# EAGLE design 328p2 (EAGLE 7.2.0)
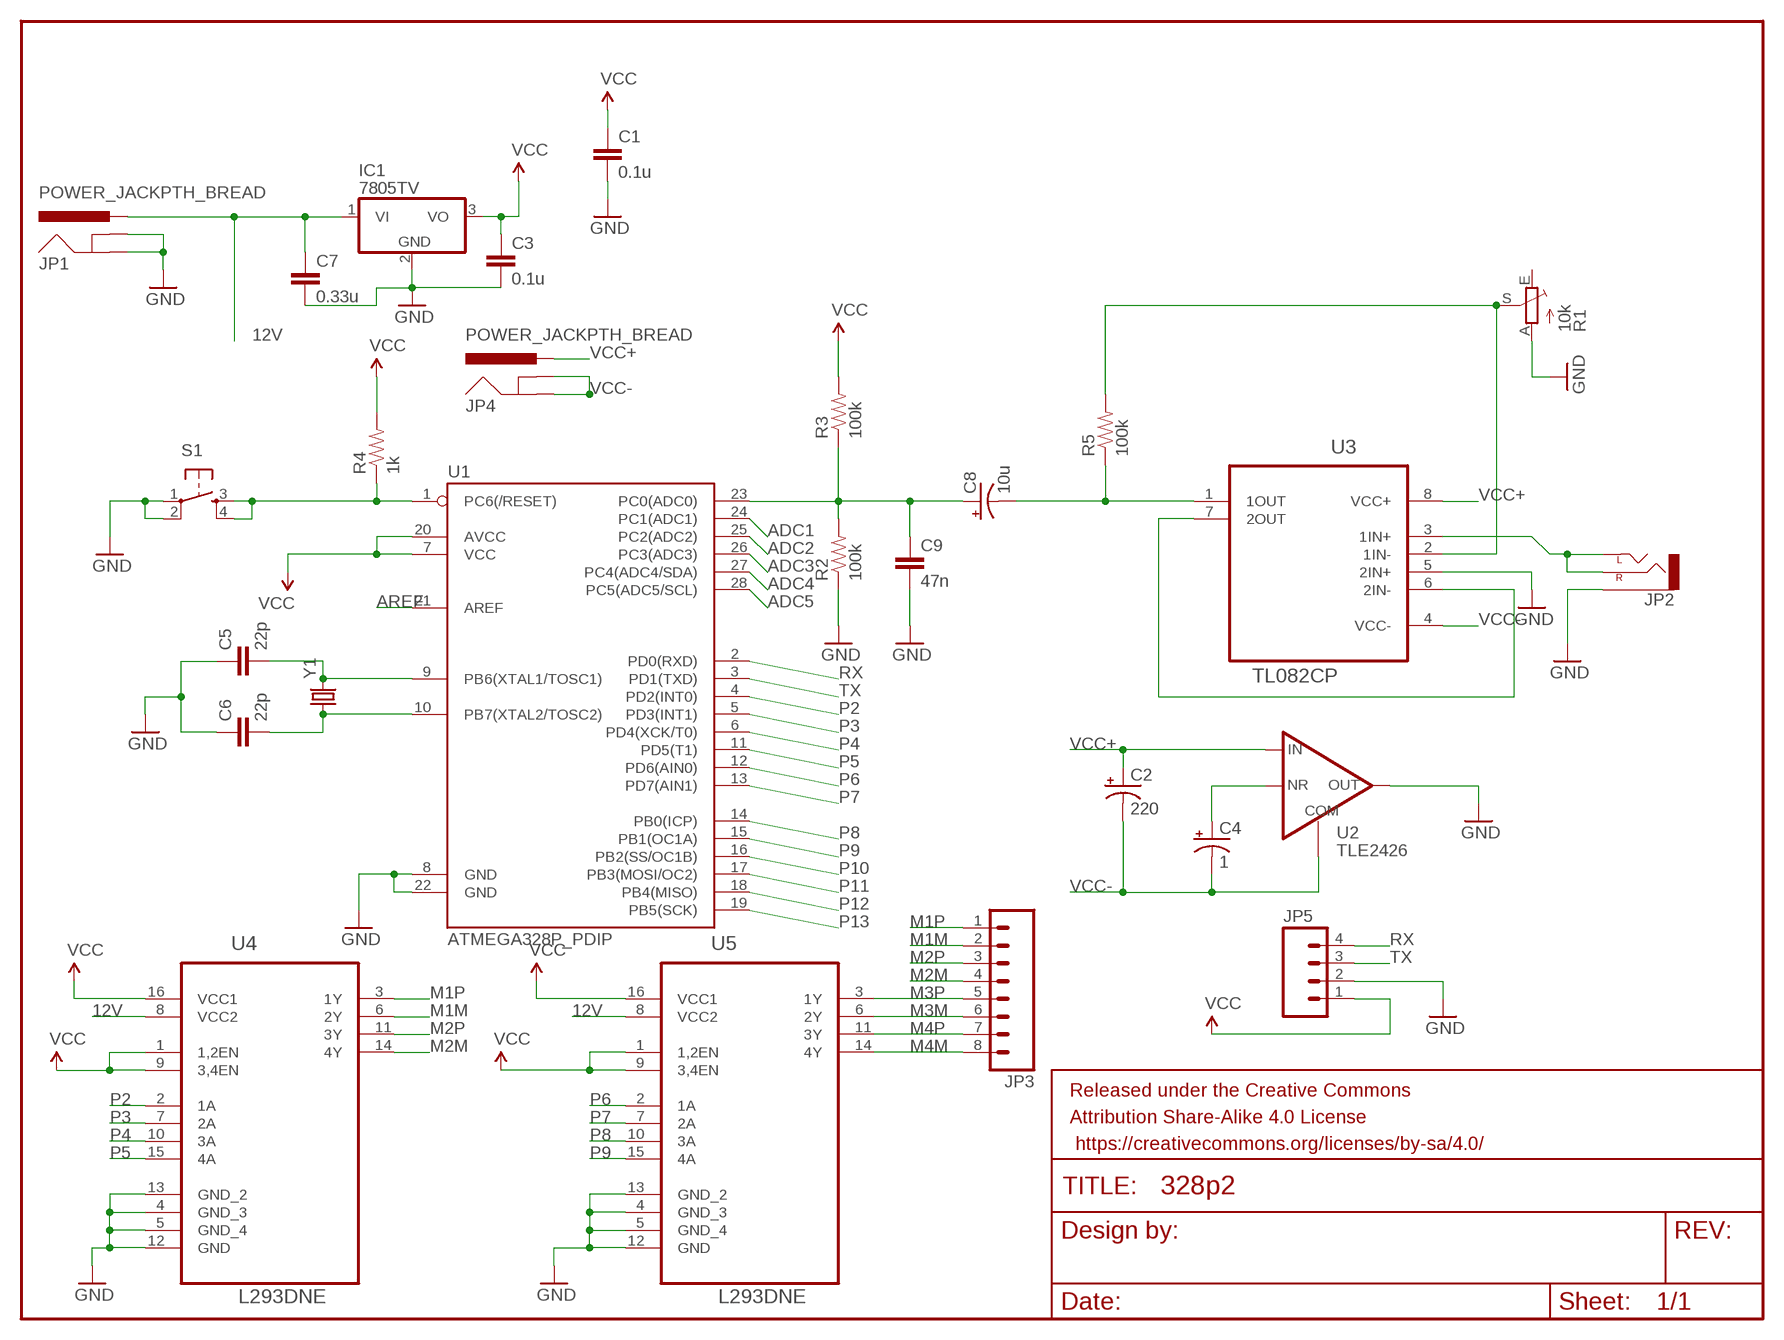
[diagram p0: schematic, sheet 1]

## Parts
C1  0.1u  CAP_  [AXIAL-5MM]
C2  220  CAP_POLPTH2  [CPOL-RADIAL-10UF-25V]
C3  0.1u  CAP_  [AXIAL-5MM]
C4  1  CAP_POLPTH1  [CPOL-RADIAL-100UF-25V]
C5  22p  CAP_  [AXIAL-5MM]
C6  22p  CAP_  [AXIAL-5MM]
C7  0.33u  CAP_  [AXIAL-5MM]
C8  10u  CAP_POLPTH1  [CPOL-RADIAL-100UF-25V]
C9  47n  CAP_  [AXIAL-5MM]
FRAME1  FRAME-LETTER  [CREATIVE_COMMONS]
IC1  7805TV  [TO220V]
JP1  POWER_JACKPTH_BREAD  [POWER_JACK_PTH_BREAD]
JP2  AUDIO-JACKPTH  [AUDIO-JACK]
JP3  M08  [1X08_ROUND]
JP4  POWER_JACKPTH_BREAD  [POWER_JACK_PTH_BREAD]
JP5  M04PTH  [1X04]
R1  10k  TRIM_EU-B25P  [B25P]
R2  100k  RESISTORPTH-1/4W  [AXIAL-0.4]
R3  100k  RESISTORPTH-1/4W  [AXIAL-0.4]
R4  1k  RESISTORPTH-1/4W  [AXIAL-0.4]
R5  100k  RESISTORPTH-1/4W  [AXIAL-0.4]
S1  TAC_SWITCHPTH  [TACTILE-PTH]
U1  ATMEGA328P_PDIP  [DIL28-3]
U2  TLE2426  TLE2426_RAIL_SPLITTER  [SO08]
U3  TL082CP  [DIP254P762X508-8]
U4  L293DNE  [DIP254P762X508-16]
U5  L293DNE  [DIP254P762X508-16]
Y1  CRYSTALHC49US  [HC49US]

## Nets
12V: C7.P$1 IC1.1(VI) JP1.PWR U4.8(VCC2) U5.8(VCC2)
ADC1: U1.24(PC1(ADC1))
ADC2: U1.25(PC2(ADC2))
ADC3: U1.26(PC3(ADC3))
ADC4: U1.27(PC4(ADC4/SDA))
ADC5: U1.28(PC5(ADC5/SCL))
AREF: U1.21(AREF)
GND: C1.P$2 C3.P$2 C5.P$1 C6.P$1 C7.P$2 C9.P$2 IC1.2(GND) JP1.GND JP1.GNDBREAK JP2.SLEEVE JP5.2 R1.A R2.P$1 S1.1 S1.2 U1.8(GND) U1.22(GND) U2.1(OUT) U3.5(2IN+) U4.4(GND_3) U4.5(GND_4) U4.12(GND) U4.13(GND_2) U5.4(GND_3) U5.5(GND_4) U5.12(GND) U5.13(GND_2)
M1M: JP3.2 U4.6(2Y)
M1P: JP3.1 U4.3(1Y)
M2M: JP3.4 U4.14(4Y)
M2P: JP3.3 U4.11(3Y)
M3M: JP3.6 U5.6(2Y)
M3P: JP3.5 U5.3(1Y)
M4M: JP3.8 U5.14(4Y)
M4P: JP3.7 U5.11(3Y)
N$1: R4.P$1 S1.3 S1.4 U1.1(PC6(/RESET))
N$2: C5.P$2 U1.9(PB6(XTAL1/TOSC1)) Y1.2
N$3: C6.P$2 U1.10(PB7(XTAL2/TOSC2)) Y1.1
N$4: R1.S R5.P$2 U3.2(1IN-)
N$5: C8.1(+) C9.P$1 R2.P$2 R3.P$1 U1.23(PC0(ADC0))
N$6: C8.2(-) R5.P$1 U3.1(1OUT)
N$7: JP2.RING(RIGHT) JP2.TIP(LEFT) U3.3(1IN+)
N$8: U3.6(2IN-) U3.7(2OUT)
N$9: C4.1(+) U2.8(NR)
P2: U1.4(PD2(INT0)) U4.2(1A)
P3: U1.5(PD3(INT1)) U4.7(2A)
P4: U1.6(PD4(XCK/T0)) U4.10(3A)
P5: U1.11(PD5(T1)) U4.15(4A)
P6: U1.12(PD6(AIN0)) U5.2(1A)
P7: U1.13(PD7(AIN1)) U5.7(2A)
P8: U1.14(PB0(ICP)) U5.10(3A)
P9: U1.15(PB1(OC1A)) U5.15(4A)
P10: U1.16(PB2(SS/OC1B))
P11: U1.17(PB3(MOSI/OC2))
P12: U1.18(PB4(MISO))
P13: U1.19(PB5(SCK))
RX: JP5.4 U1.2(PD0(RXD))
TX: JP5.3 U1.3(PD1(TXD))
VCC: C1.P$1 C3.P$1 IC1.3(VO) JP5.1 R3.P$2 R4.P$2 U1.7(VCC) U1.20(AVCC) U4.1(1,2EN) U4.9(3,4EN) U4.16(VCC1) U5.1(1,2EN) U5.9(3,4EN) U5.16(VCC1)
VCC+: C2.1(+) JP4.PWR U2.3(IN) U3.8(VCC+)
VCC-: C2.2(-) C4.2(-) JP4.GND JP4.GNDBREAK U2.2(COM) U3.4(VCC-)
Unconnected: R1.E

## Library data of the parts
C1 C3 C5-C7 C9 = SparkFun-Capacitors:CAP: Capacitor
C2 C4 C8 = SparkFun-Passives:CAP_POL: Capacitor Polarized
FRAME1 = SparkFun-Aesthetics:FRAME-LETTER: Schematic Frame; DESIGNER: NAME; VERSION: v01
IC1 = linear:78*: Positive VOLTAGE REGULATOR Source: http://cache.national.com/ds/LM/LM78L05.pdf http://www.fairchildsemi.com/ds/LM/LM7805.pdf
JP1 JP4 = SparkFun-Connectors:POWER_JACK: Power Jack This is the standard 5.5mm barrel jack for power. The PTH is the most common, proven, reliable, footprint. The Slot footprint only works if the mill layer is transmitted to the PCB fab house so be warned. Mating wall wart : TOL-00298 (and others); PROD_ID: PRT-10811
JP2 = SparkFun-Connectors:AUDIO-JACK: 3.5mm Audio Jack Simple 3.5mm common PCB mount audio jack. Variant PTH is our storefront SKU PRT-08032
JP3 = SparkFun-Connectors:M08: Header 8 Standard 8-pin 0.1" header. Use with straight break away headers (SKU : PRT-00116), right angle break away headers (PRT-00553), swiss pins (PRT-00743), machine pins (PRT-00117), and female headers (PRT-00115).
JP5 = SparkFun-Connectors:M04: Header 4 Standard 4-pin 0.1" header. Use with straight break away headers (SKU : PRT-00116), right angle break away headers (PRT-00553), swiss pins (PRT-00743), machine pins (PRT-00117), and female headers (PRT-00115). Molex polarized connector foot print use with SKU : PRT-08231 with associated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
R1 = pot:TRIM_EU-: POTENTIOMETER
R2-R5 = SparkFun-Resistors:RESISTOR: Resistor
S1 = SparkFun-Retired:TAC_SWITCH: Momentary Switch Button commonly used for reset or general input. Spark Fun Electronics SKU : COM-00097 SMT- SWCH-08247
U1 = SparkFun-DigitalIC:ATMEGA328P_PDIP: uC used in the Arduino 32kb flash, 1k EEPROM, 2k SRAM This is the through-hole version of this chip.
U2 = SparkFun-PowerIC:TLE2426_RAIL_SPLITTER; PROD_ID: VREG-12334
U3 = Texas Instruments_By_element14_Batch_1:TL082CP: OPERATIONAL AMPLIFIER; MPN: TL082CP; OC_FARNELL: 1106017; OC_NEWARK: 60K6991; PACKAGE: PDIP; SUPPLIER: Texas Instruments
U4 U5 = Texas Instruments_By_element14_Batch_1:L293DNE: QUADRUPLE HALF-H DRIVERS; MPN: L293DNE; OC_FARNELL: 1470423; OC_NEWARK: 06F9523; PACKAGE: PDIP-16; SUPPLIER: Texas Instruments
Y1 = SparkFun-FreqCtrl:CRYSTAL: Various standard crystals. Proven footprints.

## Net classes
0 default: clearance 0.205 mm

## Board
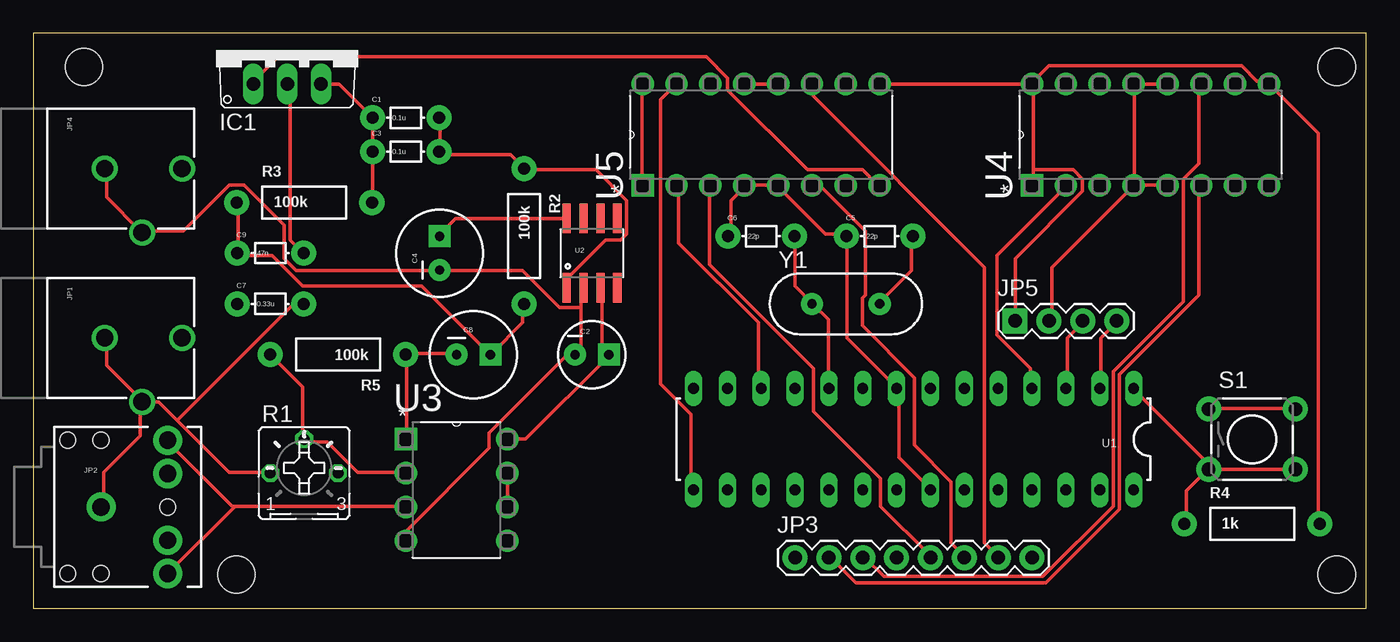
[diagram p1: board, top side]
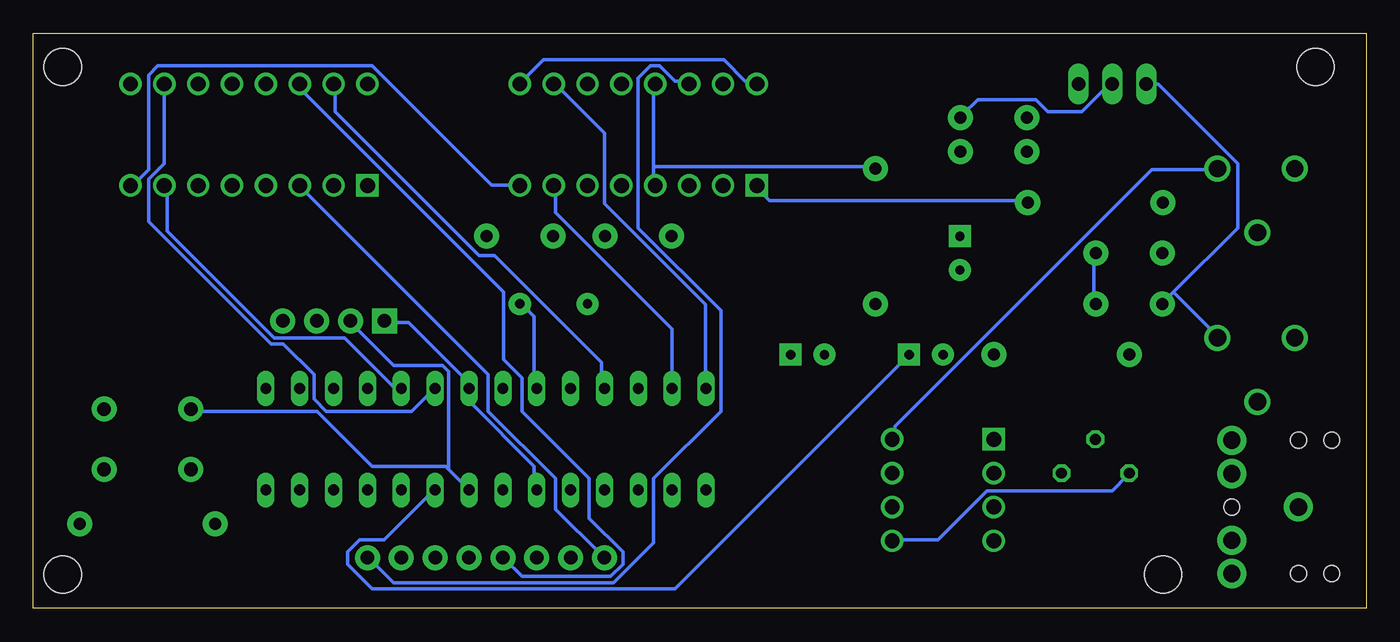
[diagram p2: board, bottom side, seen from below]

Size 100 x 43.17 mm. Coordinates in mm from the lower left corner, seen from the top.
Outline: 0,0 100,0 100,43.17 0,43.17 0,0
Copper layers (1*16): Top 0.035mm / dielectric 1.5mm / Bottom 0.035mm
Design rules "default": minimum track width 10mil, minimum drill 24mil, track to track 8mil, track to pad 8mil, pad to pad 8mil, via to via 8mil, smd to smd 8mil, copper to edge 40mil, drill to drill 8mil, minimum pad ring 10mil, minimum via ring 8mil, stop-mask expansion 4mil, vias tented up to drill 0mil, thermal gap 10mil
Holes 2.8 mm at 3.81,40.64 97.79,40.64 97.79,2.54 15.24,2.54

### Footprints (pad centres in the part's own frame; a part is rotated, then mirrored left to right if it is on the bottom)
AXIAL-5MM = drill 0.9 pad 1.88: P$1 -2.5,0; P$2 2.5,0
CPOL-RADIAL-10UF-25V = drill 0.7 pad 1.651 square: 1 1.27,0 | drill 0.7 pad 1.651: 2 -1.27,0
CPOL-RADIAL-100UF-25V = drill 0.7 pad 1.651 square: 1 1.27,0 | drill 0.7 pad 1.651: 2 -1.27,0
TO220V = drill 1.016 long: 1 -2.54,-2.54; 2 0,-2.54; 3 2.54,-2.54
POWER_JACK_PTH_BREAD = drill 1.3: GND 0,7.9; GNDBREAK 4.8,10.7; PWR 0,13.7
AUDIO-JACK = drill 1.3 pad 2.184: RING 5,5; RSH 5,2.5; SLEEVE 0,0; TIP 5,-5; TSH 5,-2.5 | hole 1.2: 0,5; -2.5,5; -2.5,-5; 0,-5; 5,0
1X08_ROUND = drill 1.016 pad 1.88: 1 0,0; 2 2.54,0; 3 5.08,0; 4 7.62,0; 5 10.16,0; 6 12.7,0; 7 15.24,0; 8 17.78,0
1X04 = drill 1.016 pad 1.88 square: 1 0,0 | drill 1.016 pad 1.88: 2 2.54,0; 3 5.08,0; 4 7.62,0
B25P = drill 0.813 octagon: A -2.54,0; E 2.54,0; S 0,2.54
AXIAL-0.4 = drill 0.9 pad 1.88: P$1 -5.08,0; P$2 5.08,0
TACTILE-PTH = drill 1.016 pad 1.88: 1 -3.251,2.261; 2 3.251,2.261; 3 -3.251,-2.261; 4 3.251,-2.261
DIL28-3 = drill 0.813 long: 1 -16.51,-3.81; 2 -13.97,-3.81; 3 -11.43,-3.81; 4 -8.89,-3.81; 5 -6.35,-3.81; 6 -3.81,-3.81; 7 -1.27,-3.81; 8 1.27,-3.81; 9 3.81,-3.81; 10 6.35,-3.81; 11 8.89,-3.81; 12 11.43,-3.81; 13 13.97,-3.81; 14 16.51,-3.81; 15 16.51,3.81; 16 13.97,3.81; 17 11.43,3.81; 18 8.89,3.81; 19 6.35,3.81; 20 3.81,3.81; 21 1.27,3.81; 22 -1.27,3.81; 23 -3.81,3.81; 24 -6.35,3.81; 25 -8.89,3.81; 26 -11.43,3.81; 27 -13.97,3.81; 28 -16.51,3.81
SO08 = smd 0.61 x 2.21: 1 -1.905,-2.616; 2 -0.635,-2.616; 3 0.635,-2.616; 4 1.905,-2.616; 5 1.905,2.616; 6 0.635,2.616; 7 -0.635,2.616; 8 -1.905,2.616
DIP254P762X508-8 = drill 1.118 square: 1 -7.62,7.62 | drill 1.118: 2 -7.62,5.08; 3 -7.62,2.54; 4 -7.62,0; 5 0,0; 6 0,2.54; 7 0,5.08; 8 0,7.62
DIP254P762X508-16 = drill 1.118 square: 1 -7.62,17.78 | drill 1.118: 2 -7.62,15.24; 3 -7.62,12.7; 4 -7.62,10.16; 5 -7.62,7.62; 6 -7.62,5.08; 7 -7.62,2.54; 8 -7.62,0; 9 0,0; 10 0,2.54; 11 0,5.08; 12 0,7.62; 13 0,10.16; 14 0,12.7; 15 0,15.24; 16 0,17.78
HC49US = drill 0.7 pad 1.651: 1 -2.54,0; 2 2.54,0

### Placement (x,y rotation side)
C1  27.94,36.83 0 top
C2  41.91,19.05 0 top
C3  27.94,34.29 0 top
C4  30.48,26.67 90 top
C5  63.5,27.94 0 top
C6  54.61,27.94 0 top
C7  17.78,22.86 0 top
C8  33.02,19.05 0 top
C9  17.78,26.67 0 top
FRAME1  not placed on the board
IC1  19.05,41.91 0 top
JP1  -2.54,20.32 270 top
JP2  5.08,7.62 0 top
JP3  57.15,3.81 0 top
JP4  -2.54,33.02 270 top
JP5  73.66,21.59 0 top
R1  20.32,10.16 0 top
R2  36.83,27.94 270 top
R3  20.32,30.48 0 top
R4  91.44,6.35 0 top
R5  22.86,19.05 180 top
S1  91.44,12.7 0 top
U1  66.04,12.7 180 top
U2  41.91,26.67 0 top
U3  35.56,5.08 0 top
U4  92.71,39.37 90 top
U5  63.5,39.37 90 top
Y1  60.96,22.86 0 top

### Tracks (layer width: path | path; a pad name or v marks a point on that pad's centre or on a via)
12V
  Top 0.254: IC1.1 16.52,39.58 18.36,41.42 50.49,41.42 52.1,39.81 52.1,38.89 58.06,32.93 62.19,32.93 63.34,31.78 U5.8
  Bottom 0.254: 14.46,23.75 15.15,23.06 C7.P$1 | 14.46,23.75 9.64,28.57 9.64,33.38 15.61,39.35 16.29,39.35 IC1.1 | 14.46,23.75 11.24,20.53 JP1.PWR | U5.8 63.57,31.78 65.64,31.78 74.59,40.73 90.65,40.73 91.34,40.04 91.34,32.93 92.49,31.78 U4.8
GND
  Top 0.254: IC1.2 19.28,39.35 19.28,27.65 20.2,26.73 C9.P$2 | C1.P$2 30.52,36.83 30.52,34.3 C3.P$2 30.52,34.07 35.8,34.07 36.72,33.15 R2.P$1 36.95,32.93 42.23,32.93 44.52,30.63 44.52,28.11 44.06,27.65 42.92,27.65 40.16,24.89 40.16,24.2 U2.1 | 10.79,14.11 9.41,15.48 8.26,15.48 JP1.GNDBREAK | 10.79,14.11 14.69,10.21 17.67,10.21 R1.A | JP1.GND 5.51,20.3 5.51,18.24 8.03,15.71 JP1.GNDBREAK | JP2.SLEEVE 5.28,7.68 5.28,10.21 8.03,12.96 8.03,15.48 JP1.GNDBREAK | 10.79,14.11 19.51,22.83 20.2,22.83 C7.P$2 | 82.62,39.35 84.92,39.35 U4.12 | 82.62,31.78 84.92,31.78 U4.5 | JP5.2 76.42,21.68 76.42,25.58 82.39,31.55 U4.4 82.62,31.78 | 82.62,31.78 82.62,39.35 | 82.62,39.35 U4.13 | U5.13 53.47,39.35 55.77,39.35 U5.12 | C6.P$1 52.33,28.11 52.33,30.63 53.24,31.55 U5.4 53.47,31.78 55.77,31.78 U5.5 56,31.55 59.44,28.11 60.82,28.11 C5.P$1 61.05,27.88 61.05,20.3 64.72,16.63 U1.8 64.95,16.4 64.95,11.35 67.24,9.06 U1.22 | S1.1 88.36,15.02 94.55,15.02 S1.2
  Bottom 0.254: C7.P$2 20.43,23.06 20.43,26.5 C9.P$2 | IC1.2 19.28,39.35 21.34,37.29 23.87,37.29 24.79,38.2 29.15,38.2 30.29,37.06 C1.P$2 | U3.5 35.34,5.16 32.13,5.16 28.46,8.83 19.05,8.83 17.9,9.97 R1.A | 53.47,33.15 53.47,31.78 U5.4 | 53.47,33.15 53.47,39.35 U5.13 | 68.85,10.43 67.47,9.06 U1.22 | 68.85,10.43 69.08,10.66 74.59,10.66 78.72,14.8 88.13,14.8 S1.1 | 68.85,10.43 68.85,17.78 69.31,18.24 72.98,18.24 76.19,21.45 JP5.2 | 53.47,33.15 36.95,33.15 R2.P$1
M1M
  Top 0.254: U4.6 87.44,31.55 87.44,23.52 81.47,17.55 81.47,7.45 75.97,1.94 61.74,1.94 59.9,3.78 JP3.2
M1P
  Bottom 0.254: U4.3 79.87,31.55 65.87,17.55 65.87,14.8 60.82,9.75 60.82,7.45 57.38,4.01 JP3.1
M2M
  Bottom 0.254: U4.14 79.87,39.35 79.87,38.89 64.72,23.75 64.72,18.7 63.34,17.32 63.34,14.8 58.29,9.75 58.29,6.76 55.77,4.24 55.77,3.32 56.69,2.4 63.34,2.4 64.72,3.78 JP3.4
M2P
  Top 0.254: U4.11 87.44,39.35 87.44,33.38 86.29,32.24 86.29,23.06 81.01,17.78 81.01,7.68 75.73,2.4 63.8,2.4 62.42,3.78 JP3.3
M3M
  Top 0.254: U5.6 58.52,31.55 59.21,31.55 62.42,28.34 62.42,23.52 62.19,23.29 62.19,21.22 66.1,17.32 66.1,12.27 68.85,9.52 68.85,4.93 69.77,4.01 JP3.6
M3P
  Top 0.254: U5.3 50.72,31.55 50.72,25.81 58.52,18.01 58.52,14.8 63.57,9.75 63.57,7.68 67.24,4.01 JP3.5
M4M
  Bottom 0.254: U5.14 50.95,39.58 51.87,39.58 53.01,40.73 53.7,40.73 54.62,39.81 54.62,28.57 48.42,22.37 48.42,14.8 53.47,9.75 53.47,4.93 56.46,1.94 72.98,1.94 74.82,3.78 JP3.8
M4P
  Top 0.254: U5.11 58.52,39.35 58.52,38.43 71.37,25.58 71.37,4.93 72.29,4.01 JP3.7
N$1
  Top 0.254: U1.1 82.62,16.4 88.36,10.66 S1.3 | R4.P$1 86.52,6.53 86.52,8.83 88.13,10.43 S1.3 | S1.4 94.55,10.43 88.36,10.43 S1.3
N$2
  Top 0.254: C5.P$2 65.87,27.88 65.87,25.35 63.57,23.06 Y1.2
  Bottom 0.254: U1.9 62.42,16.63 62.42,21.91 63.34,22.83 Y1.2
N$3
  Top 0.254: U1.10 59.67,16.63 59.67,21.68 58.52,22.83 Y1.1 58.29,23.06 57.15,24.2 57.15,27.88 C6.P$2
N$4
  Top 0.254: R5.P$2 17.9,18.93 20.2,16.63 20.2,12.73 R1.S 20.43,12.5 22.03,12.5 24.33,10.21 27.77,10.21 U3.2
N$5
  Top 0.254: R3.P$1 15.38,30.4 15.38,26.73 C9.P$1 15.38,26.5 17.9,26.5 20.2,24.2 29.15,24.2 34.2,19.16 C8.1 34.42,19.16 36.72,21.45 36.72,22.83 R2.P$2
  Bottom 0.254: U1.23 70,8.83 73.67,5.16 75.5,5.16 76.42,4.24 76.42,3.32 74.59,1.48 51.87,1.48 34.42,18.93 C8.1
N$6
  Top 0.254: C8.2 31.67,19.16 28,19.16 R5.P$1 28,18.93 28,12.73 U3.1
N$7
  Top 0.254: 15.15,7.68 14.92,7.68 10.1,12.5 JP2.RING | 15.15,7.68 27.77,7.68 U3.3 | 15.15,7.68 10.1,2.63 JP2.TIP
N$8
  Top 0.254: U3.6 35.57,7.68 35.57,9.97 U3.7
N$9
  Top 0.254: U2.8 39.93,29.25 31.67,29.25 30.52,28.11 C4.1
P2
  Top 0.254: U1.4 74.82,16.63 74.82,18.01 72.29,20.53 72.29,26.5 77.34,31.55 U4.2
P3
  Bottom 0.254: U1.5 72.52,16.63 72.98,16.63 76.65,20.3 81.93,20.3 89.96,28.34 89.96,31.55 U4.7
P4
  Bottom 0.254: U1.6 70,16.4 71.6,14.8 78.03,14.8 78.95,15.71 78.95,17.55 81.24,19.84 82.16,19.84 91.34,29.02 91.34,32.24 90.19,33.38 90.19,39.35 U4.10
P5
  Bottom 0.254: U1.11 57.38,16.63 57.38,18.47 65.41,26.5 66.56,26.5 77.34,37.29 77.34,39.35 U4.15
P6
  Top 0.254: U1.12 54.39,16.63 54.39,21.45 48.42,27.42 48.42,31.55 U5.2
P7
  Bottom 0.254: U1.13 52.1,16.63 52.1,20.99 60.82,29.71 60.82,31.55 U5.7
P8
  Bottom 0.254: U1.14 49.57,16.63 49.57,22.83 57.15,30.4 57.15,35.68 60.82,39.35 U5.10
P9
  Top 0.254: U1.15 49.34,9.06 49.34,14.57 47.05,16.86 47.05,38.2 48.2,39.35 U5.15
RX
  Top 0.254: U1.2 80.1,16.63 80.1,20.3 81.24,21.45 JP5.4
TX
  Top 0.254: U1.3 77.57,16.63 77.57,20.3 78.72,21.45 JP5.3
VCC
  Top 0.254: R3.P$2 25.47,30.63 25.47,34.07 C3.P$1 25.47,34.3 25.47,36.83 C1.P$1 25.25,37.06 22.95,39.35 21.8,39.35 IC1.3 | U5.1 45.67,31.78 45.67,39.35 U5.16 | U5.9 63.57,39.35 74.82,39.35 U4.16 | 75.05,32.93 75.05,39.35 U4.16 | 75.05,32.93 75.05,31.78 U4.1 | U4.16 75.05,39.58 76.19,40.73 90.65,40.73 91.8,39.58 92.49,39.58 U4.9 92.72,39.35 96.39,35.68 96.39,6.53 R4.P$2 | 75.05,32.93 78.03,32.93 78.72,32.24 78.72,31.32 73.67,26.27 73.67,21.68 JP5.1
  Bottom 0.254: U1.20 62.42,9.06 62.42,10.66 67.24,15.48 67.24,16.4 U1.7 67.47,16.63 67.47,17.09 71.83,21.45 73.44,21.45 JP5.1 | U5.16 45.9,39.58 46.59,39.58 48.2,41.19 61.74,41.19 63.34,39.58 U5.9 | R3.P$2 25.47,30.63 44.75,30.63 45.67,31.55 U5.1
VCC+
  Top 0.254: U2.3 42.69,23.98 42.69,19.61 43.15,19.16 C2.1 43.15,18.93 36.95,12.73 35.57,12.73 U3.8
  Bottom 0.254: JP4.PWR 11.24,32.93 16.07,32.93 35.34,13.65 35.34,12.73 U3.8
VCC-
  Top 0.254: JP4.GND 5.51,32.93 5.51,30.86 8.03,28.34 JP4.GNDBREAK 8.26,28.34 11.24,28.34 14.69,31.78 15.84,31.78 18.82,28.79 18.82,26.27 19.74,25.35 30.29,25.35 C4.2 30.52,25.35 36.72,25.35 39.47,22.6 41.08,22.6 | 41.08,22.6 41.08,19.39 40.85,19.16 C2.2 40.62,18.93 39.93,18.93 34.2,13.19 34.2,12.04 28,5.84 28,5.16 U3.4 | 41.08,22.6 41.08,23.98 U2.2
